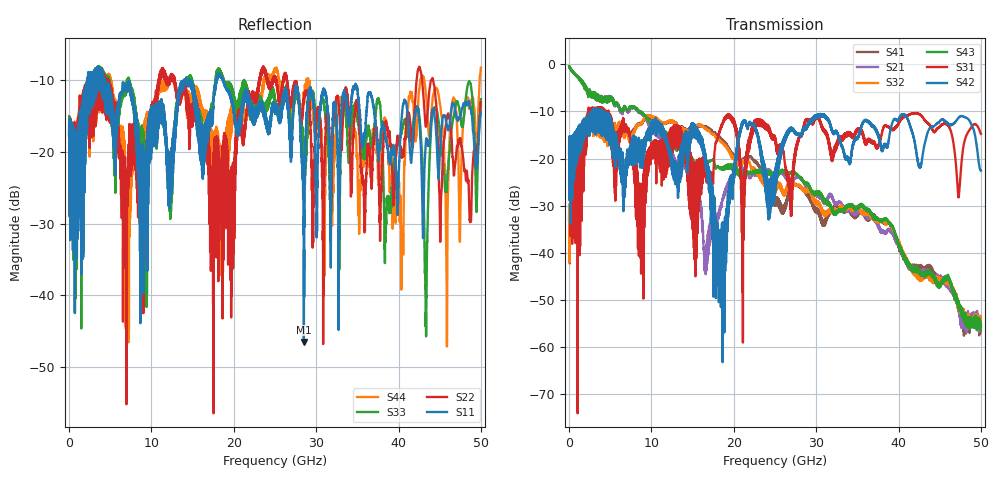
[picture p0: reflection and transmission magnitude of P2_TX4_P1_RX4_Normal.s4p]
!Keysight Technologies,N5225A,MY51441389,A.10.49.11
!Date: Monday, July 08, 2019 13:25:38
!Correction: S11(Full 4 Port(1,2,3,4))
!S12(Full 4 Port(1,2,3,4))
!S13(Full 4 Port(1,2,3,4))
!S14(Full 4 Port(1,2,3,4))
!S21(Full 4 Port(1,2,3,4))
!S22(Full 4 Port(1,2,3,4))
!S23(Full 4 Port(1,2,3,4))
!S24(Full 4 Port(1,2,3,4))
!S31(Full 4 Port(1,2,3,4))
!S32(Full 4 Port(1,2,3,4))
!S33(Full 4 Port(1,2,3,4))
!S34(Full 4 Port(1,2,3,4))
!S41(Full 4 Port(1,2,3,4))
!S42(Full 4 Port(1,2,3,4))
!S43(Full 4 Port(1,2,3,4))
!S44(Full 4 Port(1,2,3,4))
!S4P File: Measurements: <S11,S12,S13,S14>,
!<S21,S22,S23,S24>,
!<S31,S32,S33,S34>,
!<S41,S42,S43,S44>:
# Hz S  dB  R 50
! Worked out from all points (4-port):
!   5000 points, 10 MHz to 50 GHz, reference 50 ohm
!   strongest paths, dB at 10 MHz, 12.51 GHz, 25.01 GHz, 37.51 GHz, 50 GHz:
!     S42: -19.1, -21.0, -24.3, -14.7, -22.5
!     S31: -19.1, -13.6, -16.3, -17.3, -14.8
!     S43: -0.4, -16.6, -23.4, -32.9, -55.6
!     S32: -33.1, -12.2, -26.2, -33.3, -55.3
!     S21: -0.4, -18.2, -23.0, -34.0, -55.6
!     S41: -32.8, -12.2, -29.2, -33.1, -55.4
!   lowest |S11| = -46.5 dB at 28.51 GHz (marker M1), VSWR 1.01, Z = 49.5 + j0.116 ohm
!   |S11| at or under -10 dB: 4.333 GHz to 13.96 GHz (9.625 GHz wide, 105 % of centre); 14.71 GHz to 17.88 GHz (3.172 GHz wide, 19.5 % of centre); 18.69 GHz to end of sweep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
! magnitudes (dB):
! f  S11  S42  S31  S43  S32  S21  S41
! 10 MHz  -17.8  -19.1  -19.1  -0.4  -33.1  -0.4  -32.8
! 16.58 GHz  -18.3  -20.6  -22.9  -21.1  -13.7  -42.8  -13.2
! 18.39 GHz  -9.2  -45.4  -13.5  -22.1  -16.3  -30.6  -15.7
! 21.15 GHz  -12.7  -12.0  -31.4  -23.3  -20.6  -22.6  -20.1
! 28.51 GHz  -46.5  -13.7  -13.2  -24.9  -26.5  -25.0  -26.5
! 40.37 GHz  -15.3  -10.6  -11.6  -40.1  -39.7  -39.6  -40.4
! 50 GHz  -14.5  -22.5  -14.8  -55.6  -55.3  -55.6  -55.4
